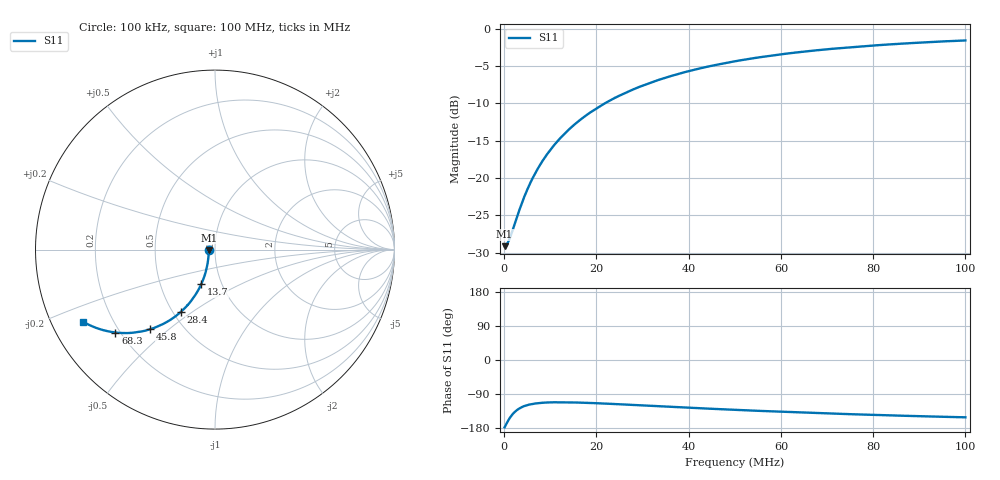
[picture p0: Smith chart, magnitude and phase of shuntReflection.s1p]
# Hz S RI R 50.0
! written by SimSmith version 18.3h
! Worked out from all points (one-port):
!   1000 points, 100 kHz to 100 MHz, reference 50 ohm
!   lowest |S11| = -29.1 dB at 100 kHz (marker M1), VSWR 1.07, Z = 46.6 - j0.139 ohm
!   |S11| at or under -10 dB: start of sweep to 21.78 MHz
!   S11 on the Smith chart (normalised r, x): 100 kHz: 0.93, -0.00; 13.7 MHz: 0.80, -0.32; 28.4 MHz: 0.55, -0.45; 45.8 MHz: 0.33, -0.43; 68.3 MHz: 0.18, -0.35; 100 MHz: 0.09, -0.25
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100000  -0.0349 -0.00149
600000  -0.0348 -0.00876
1100000  -0.035 -0.0162
1600000  -0.0354 -0.0234
3200000  -0.0373 -0.0467
4100000  -0.0387 -0.0599
5300000  -0.0413 -0.0771
6500000  -0.0445 -0.0942
7900000  -0.049 -0.1141
9300000  -0.0545 -0.1335
1.1e7  -0.0621 -0.1567
1.26e7  -0.0703 -0.1778
1.37e7  -0.0763 -0.1922
1.63e7  -0.0926 -0.2246
1.89e7  -0.111 -0.2551
2.18e7  -0.1338 -0.2867
2.51e7  -0.1619 -0.3194
2.84e7  -0.192 -0.3484
3.29e7  -0.235 -0.3822
3.76e7  -0.2812 -0.4103
4.58e7  -0.3616 -0.4437
5.01e7  -0.4024 -0.4547
5.57e7  -0.4531 -0.4627
6.26e7  -0.5108 -0.4651
6.83e7  -0.5546 -0.462
7.51e7  -0.6018 -0.4537
8.76e7  -0.6755 -0.4308
1e8  -0.7333 -0.4035
